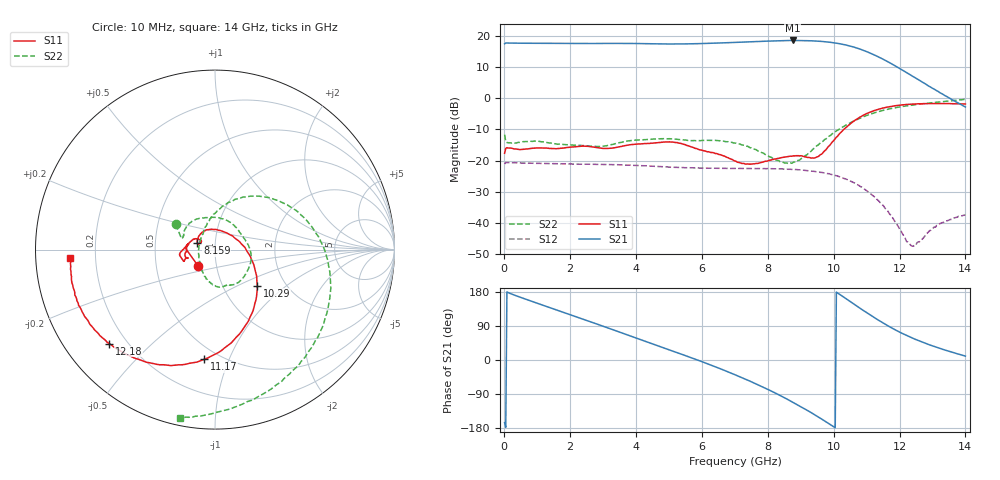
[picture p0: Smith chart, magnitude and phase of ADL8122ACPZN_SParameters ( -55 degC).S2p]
! "Analog Devices, Inc."
! Device:	ADL8122ACPZN
! Description:	"10 kHz to 10 GHz, Wideband, Low Noise Amplifier"
! Conditions:	Vdd = 5.0 V
!		IDQ = 95 mA
!		Pin = -25 dBm
!		Operating Temperature = +25 C (at package bottom)
! Product validation unit SN1 soldered down to Evaluation Board as shown on ADL8122-EVALZ User Guide. Board loss de-embedded from S21 magnitude.  All other RF measurements reference to RF coaxial connector.
! Frequency (GHz)	S11_Mag (dB)	S11_Phase (deg)	S21_Mag (dB)	S21_Phase (deg)	S12_Mag (dB)	S12_Phase (deg)	S22_Mag (dB)	S22_Phase (deg)
#  GHZ  S  DB  R 50
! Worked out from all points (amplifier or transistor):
!   401 points, 10 MHz to 14 GHz, reference 50 ohm
!   highest |S21| = 18.5 dB at 8.754 GHz (marker M1)
!   |S21| within 3 dB of that: start of sweep to 10.86 GHz
!   unconditionally stable (mu >= 1): start of sweep to end of sweep
!   at 2.318 GHz: K = 1.07, MAG = 17.7 dB, |S12| = -21.2 dB
!   at 7.005 GHz: K = 1.11, MAG = 18.2 dB, |S12| = -22.5 dB
!   at 14 GHz: K = 1.07, MAG = 15.6 dB, |S12| = -37.4 dB
!   S11 on the Smith chart (normalised r, x): 10 MHz: 0.82, -0.15; 8.159 GHz: 0.82, +0.06; 10.29 GHz: 1.45, -0.65; 11.17 GHz: 0.42, -0.82; 12.18 GHz: 0.14, -0.37; 14 GHz: 0.11, -0.03
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0.01  -17.65 -135.0  17.40 -165.2  -21.07 15.8  -11.69 147.3
0.1499  -15.98 171.9  17.64 176.7  -20.66 -2.7  -14.28 160.8
0.91935  -16.00 174.8  17.57 152.3  -20.86 -21.5  -13.73 134.3
1.653825  -16.13 -176.8  17.52 129.8  -20.98 -38.5  -14.73 102.0
2.353325  -15.38 -169.7  17.48 108.7  -21.13 -55.2  -15.18 63.9
3.472525  -15.62 -163.6  17.53 74.4  -21.32 -83.3  -14.34 2.9
4.69665  -14.20 -167.6  17.37 36.1  -21.89 -116.4  -13.03 -48.7
5.95575  -16.55 165.4  17.47 -2.9  -22.37 -150.2  -13.63 -74.4
6.480375  -17.89 151.9  17.64 -20.4  -22.49 -164.9  -13.59 -84.6
7.005  -20.11 146.9  17.85 -38.9  -22.50 179.7  -14.39 -96.5
7.5646  -21.02 154.5  18.08 -59.9  -22.57 162.3  -16.27 -113.1
8.159175  -19.60 159.7  18.32 -84.2  -22.60 142.9  -19.33 -141.9
8.75375  -18.55 135.0  18.47 -111.2  -22.81 121.3  -20.71 159.1
9.348325  -19.13 74.9  18.35 -140.5  -23.38 97.5  -16.58 107.2
9.837975  -15.52 4.0  17.94 -167.0  -24.19 75.4  -12.33 80.9
10.29265  -10.16 -40.5  17.20 166.8  -25.64 53.1  -9.13 57.8
10.74733  -6.42 -71.9  15.90 139.7  -27.84 29.2  -6.66 33.5
11.16703  -4.24 -95.6  14.16 115.6  -30.99 6.1  -4.97 10.6
11.69165  -2.73 -120.3  11.39 88.0  -37.00 -25.1  -3.44 -16.8
12.1813  -2.06 -138.4  8.40 66.1  -45.09 -78.3  -2.52 -39.2
12.95075  -1.71 -157.8  3.50 38.8  -42.34 165.7  -1.50 -69.2
14  -1.86 -176.5  -2.83 10.2  -37.40 131.0  -0.37 -101.8
